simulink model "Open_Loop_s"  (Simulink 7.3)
settings: Solver=ode45  StartTime=0.0  StopTime=10  FixedStep=0.04  RelTol=1e-3
undefined symbols (not defined in the file or in its folder): Acs, Av1, Bcs, Bv1, Ccs, Cv1, Dcs, Dv1

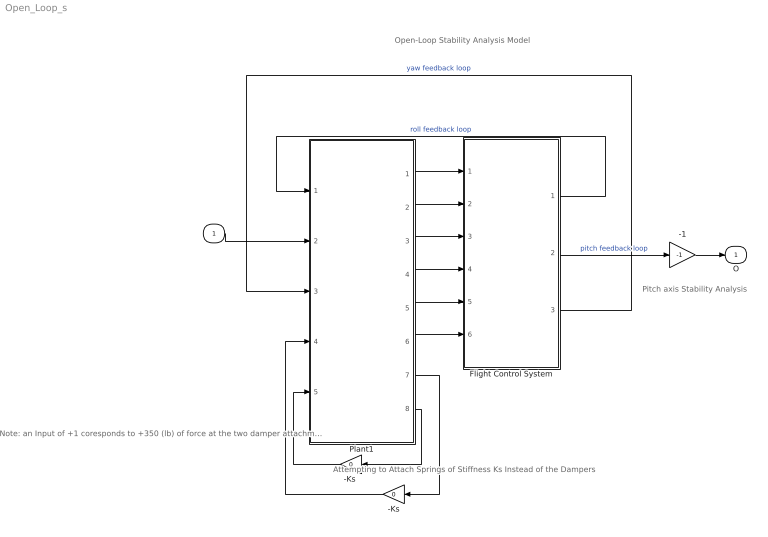
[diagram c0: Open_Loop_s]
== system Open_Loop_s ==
  note: Open-Loop Stability Analysis Model
  note: Attempting to Attach Springs of Stiffness Ks Instead of the Dampers
  note: Pitch axis Stability Analysis
  note: Note: an Input of +1 coresponds to +350 (lb) of force at the two damper attachments because the vehicle model force inputs are normalized at 350 lb
  I : Inport  OutDataType=sfix(16)  OutScaling=2^0
  -1 : Gain  Gain=-1  ParameterDataType=sfix(16)  ParameterScaling=2^0  OutDataType=sfix(16)  OutScaling=2^0
  -Ks : Gain  Gain=0  ParameterDataType=sfix(16)  ParameterScaling=2^0  OutDataType=sfix(16)  OutScaling=2^0
  "-Ks " : Gain  Gain=0  ParameterDataType=sfix(16)  ParameterScaling=2^0  OutDataType=sfix(16)  OutScaling=2^0
  Flight Control System : Subsystem
  Plant1 : Subsystem
  O : Outport  OutDataType=sfix(16)  OutScaling=2^0
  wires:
  -1/1 -> O/1
  Plant1/1(phi) -> Flight Control System/1(Phi)
  Plant1/2(theta) -> Flight Control System/2(Theta)
  Plant1/3(psi) -> Flight Control System/3(Psi)
  Plant1/4(P) -> Flight Control System/4(P)
  Plant1/5(Q) -> Flight Control System/5(Q)
  Plant1/6(R) -> Flight Control System/6(R)
  -Ks/1 -> Plant1/4(F-left)
  "-Ks "/1 -> Plant1/5(F-right)
  Plant1/8(dZ-Rght) -> "-Ks "/1
  Plant1/7(dZ-Left) -> -Ks/1
  Flight Control System/3(DR-TVC) -> Plant1/3(DR)  "yaw feedback loop"
  I/1 -> Plant1/2(DQ)
  Flight Control System/2(DQ-TVC) -> -1/1  "pitch feedback loop"
  Flight Control System/1(DP-TVC) -> Plant1/1(DP)  "roll feedback loop"

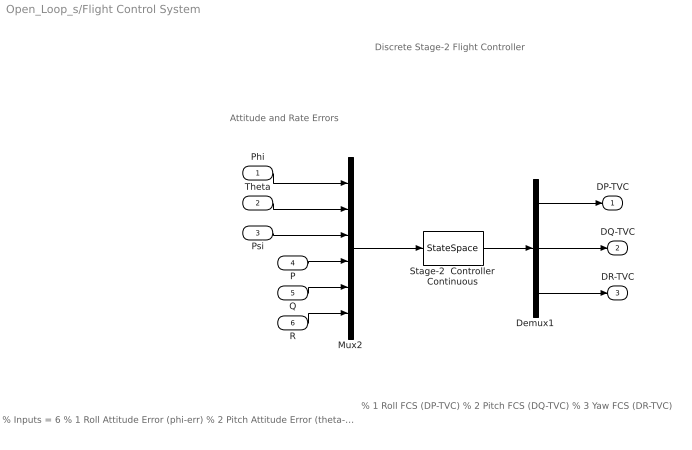
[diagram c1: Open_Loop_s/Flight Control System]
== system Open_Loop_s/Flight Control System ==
  note: Discrete Stage-2 Flight Controller
  note: Attitude and Rate Errors
  note: % Inputs = 6 % 1 Roll Attitude Error (phi-err) % 2 Pitch Attitude Error (theta-err) % 3 Yaw Attitude Error (psi-err) % 4 Roll Rate Error (p-err) % 5 Pitch Rate Error (q-err) % 6 Yaw Rate Error (r-err)
  note: % 1 Roll FCS (DP-TVC) % 2 Pitch FCS (DQ-TVC) % 3 Yaw FCS (DR-TVC)
  Phi : Inport  OutDataType=sfix(16)  OutScaling=2^0
  Theta : Inport  Port=2  OutDataType=sfix(16)  OutScaling=2^0
  Psi : Inport  Port=3  OutDataType=sfix(16)  OutScaling=2^0
  P : Inport  Port=4  OutDataType=sfix(16)  OutScaling=2^0
  Q : Inport  Port=5  OutDataType=sfix(16)  OutScaling=2^0
  R : Inport  Port=6  OutDataType=sfix(16)  OutScaling=2^0
  Demux1 : Demux  Outputs=3
  Mux2 : Mux  Inputs=6
  Stage-2  Controller Continuous : StateSpace  A=Acs  B=Bcs  C=Ccs  D=Dcs
  DP-TVC : Outport  OutDataType=sfix(16)  OutScaling=2^0
  DQ-TVC : Outport  Port=2  OutDataType=sfix(16)  OutScaling=2^0
  DR-TVC : Outport  Port=3  OutDataType=sfix(16)  OutScaling=2^0
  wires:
  Q/1 -> Mux2/5
  R/1 -> Mux2/6
  Phi/1 -> Mux2/1
  Theta/1 -> Mux2/2
  Psi/1 -> Mux2/3
  Mux2/1 -> Stage-2  Controller Continuous/1
  Stage-2  Controller Continuous/1 -> Demux1/1
  P/1 -> Mux2/4
  Demux1/2 -> DQ-TVC/1
  Demux1/1 -> DP-TVC/1
  Demux1/3 -> DR-TVC/1

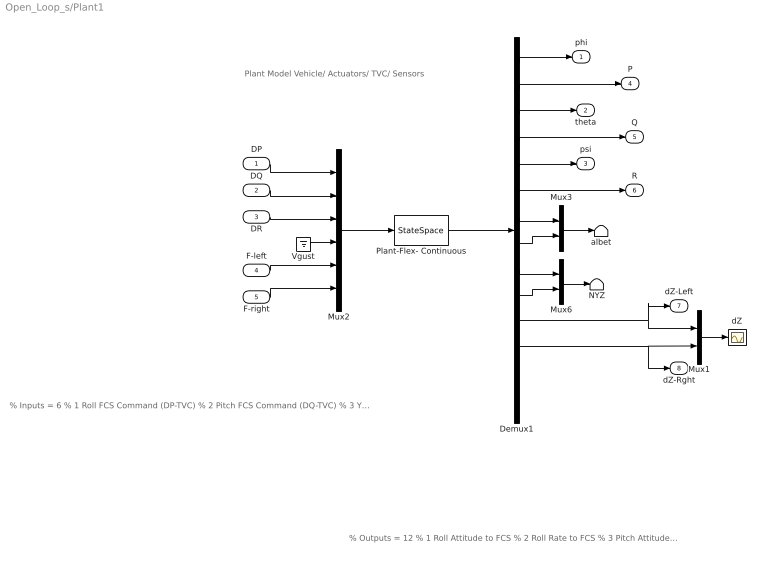
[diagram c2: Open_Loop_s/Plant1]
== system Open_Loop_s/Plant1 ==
  note: Plant Model Vehicle/ Actuators/ TVC/ Sensors
  note: % Inputs = 6 % 1 Roll FCS Command (DP-TVC) % 2 Pitch FCS Command (DQ-TVC) % 3 Yaw FCS Command (DR-TVC) % 4 Wind-Gust Velocity (ft/sec) % 5 Left Coulomb Damper Force % 6 Right Coulomb Damper Force
  note: % Outputs = 12 % 1 Roll Attitude to FCS % 2 Roll Rate to FCS % 3 Pitch Attitude to FCS % 4 Pitch Rate to FCS % 5 Yaw Attitude to FCS % 6 Yaw Rate to FCS % 7 Angle of Attack, alpha (rad) % 8 Angle of Sideslip, beta (rad) % 9 Normal Accelerometer, Nz (ft/sec^2) % 10 Lateral Accelerometer, Ny (ft/sec^2) % 11 Left Damper Extension (ft) % 12 Right Damper Extension (ft) % 13 Left Damper Rate (ft/sec) % 14 Right Damper Rate (ft/s)
  DP : Inport  OutDataType=sfix(16)  OutScaling=2^0
  DQ : Inport  Port=2  OutDataType=sfix(16)  OutScaling=2^0
  DR : Inport  Port=3  OutDataType=sfix(16)  OutScaling=2^0
  F-left : Inport  Port=4  OutDataType=sfix(16)  OutScaling=2^0
  F-right : Inport  Port=5  OutDataType=sfix(16)  OutScaling=2^0
  Demux1 : Demux  Outputs=14
  Mux1 : Mux  Inputs=2
  Mux2 : Mux  Inputs=6
  Mux3 : Mux  Inputs=2
  Mux6 : Mux  Inputs=2
  NYZ : Terminator
  Plant-Flex- Continuous : StateSpace  A=Av1  B=Bv1  C=Cv1  D=Dv1
  Vgust : Ground
  albet : Terminator
  dZ : Scope
  phi : Outport  OutDataType=sfix(16)  OutScaling=2^0
  theta : Outport  Port=2  OutDataType=sfix(16)  OutScaling=2^0
  psi : Outport  Port=3  OutDataType=sfix(16)  OutScaling=2^0
  P : Outport  Port=4  OutDataType=sfix(16)  OutScaling=2^0
  Q : Outport  Port=5  OutDataType=sfix(16)  OutScaling=2^0
  R : Outport  Port=6  OutDataType=sfix(16)  OutScaling=2^0
  dZ-Left : Outport  Port=7  OutDataType=sfix(16)  OutScaling=2^0
  dZ-Rght : Outport  Port=8  OutDataType=sfix(16)  OutScaling=2^0
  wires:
  F-left/1 -> Mux2/5
  F-right/1 -> Mux2/6
  DP/1 -> Mux2/1
  DQ/1 -> Mux2/2
  DR/1 -> Mux2/3
  Demux1/7 -> Mux3/1
  Demux1/9 -> Mux6/1
  Demux1/11 -> dZ-Left/1, Mux1/1
  Demux1/12 -> dZ-Rght/1, Mux1/2
  Mux2/1 -> Plant-Flex- Continuous/1
  Mux3/1 -> albet/1
  Mux6/1 -> NYZ/1
  Vgust/1 -> Mux2/4
  Demux1/2 -> P/1
  Demux1/6 -> R/1
  Demux1/8 -> Mux3/2
  Demux1/10 -> Mux6/2
  Plant-Flex- Continuous/1 -> Demux1/1
  Mux1/1 -> dZ/1
  Demux1/3 -> theta/1
  Demux1/1 -> phi/1
  Demux1/5 -> psi/1
  Demux1/4 -> Q/1
